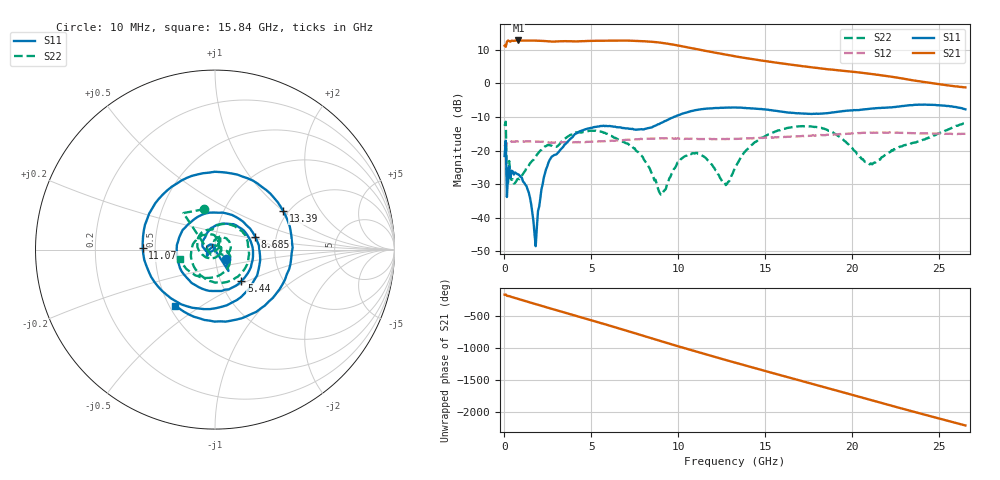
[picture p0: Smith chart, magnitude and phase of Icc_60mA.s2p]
!Keysight Technologies,N5245A,MY52451697,A.10.60.06
!Date: Thursday, May 06, 2021 15:05:40
!Correction: S11(Full 2 Port(1,4))
!S41(Full 2 Port(1,4))
!S14(Full 2 Port(1,4))
!S44(Full 2 Port(1,4))
!S2P File: Measurements: S11, S41, S14, S44:
# Hz S  dB  R 50
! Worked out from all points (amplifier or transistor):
!   401 points, 10 MHz to 26.5 GHz, reference 50 ohm
!   highest |S21| = 12.8 dB at 804.7 MHz (marker M1)
!   |S21| within 3 dB of that: start of sweep to 11.46 GHz
!   unconditionally stable (mu >= 1): start of sweep to end of sweep
!   at 4.381 GHz: K = 1.13, MAG = 12.9 dB, |S12| = -17.5 dB
!   at 13.26 GHz: K = 1.23, MAG = 9.4 dB, |S12| = -16.5 dB
!   at 26.5 GHz: K = 2.49, MAG = 0.1 dB, |S12| = -15.0 dB
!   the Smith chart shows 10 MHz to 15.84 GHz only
!   S11 on the Smith chart (normalised r, x): 10 MHz: 1.13, -0.12; 5.44 GHz: 1.25, -0.46; 8.685 GHz: 1.56, +0.24; 11.07 GHz: 0.43, +0.01; 13.39 GHz: 1.88, +1.00; 15.84 GHz: 0.54, -0.39
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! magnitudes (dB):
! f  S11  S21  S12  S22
! 10 MHz  -21.6  11.3  -18.3  -12.6
! 274.9 MHz  -24.7  12.7  -17.4  -23.1
! 804.7 MHz  -27.1  12.8  -17.3  -28.4
! 1.335 GHz  -31.7  12.8  -17.3  -25.0
! 1.798 GHz  -48.5  12.8  -17.3  -21.9
! 2.262 GHz  -28.1  12.7  -17.5  -19.1
! 2.593 GHz  -22.9  12.5  -17.6  -18.4
! 4.447 GHz  -14.1  12.6  -17.5  -14.6
! 5.44 GHz  -12.8  12.7  -17.2  -14.3
! 7.427 GHz  -13.7  12.7  -16.7  -19.3
! 8.685 GHz  -12.6  12.3  -16.4  -28.7
! 8.884 GHz  -12.1  12.2  -16.4  -32.2
! 10.08 GHz  -9.3  11.2  -16.5  -23.3
! 11.07 GHz  -7.9  10.2  -16.5  -20.7
! 12.66 GHz  -7.2  8.7  -16.6  -29.5
! 13.26 GHz  -7.2  8.1  -16.5  -25.3
! 13.39 GHz  -7.2  8.0  -16.5  -24.0
! 15.84 GHz  -8.3  6.1  -16.1  -14.0
! 17.69 GHz  -9.1  4.8  -15.5  -12.9
! 20.87 GHz  -7.6  3.0  -14.7  -23.9
! 22.13 GHz  -7.2  2.1  -14.6  -20.5
! 26.5 GHz  -7.7  -1.2  -15.0  -11.8
